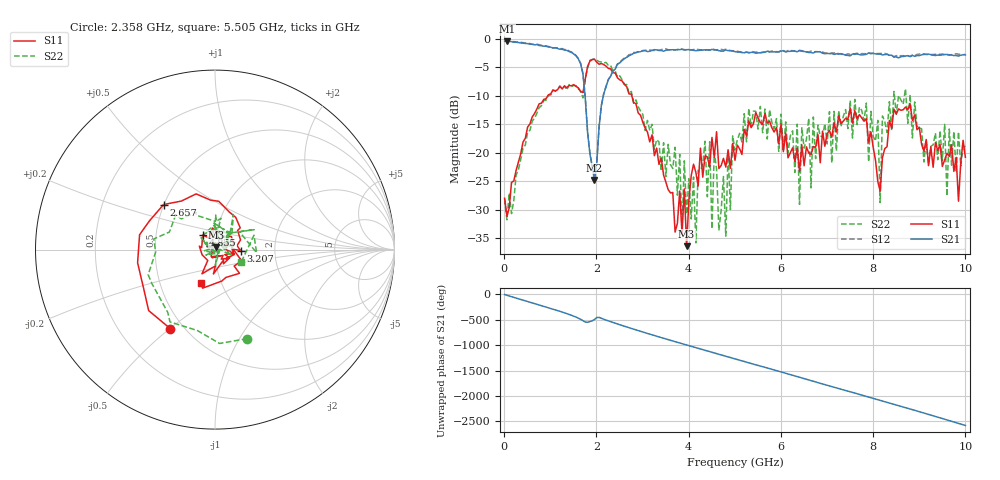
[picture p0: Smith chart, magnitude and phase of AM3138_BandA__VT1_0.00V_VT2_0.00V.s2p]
! Date/Time: Tue, Nov 13, 2018 4:41 PM
! Network Analyzer: Agilent Technologies E8364B Rev: A.07.50.67
! Sweep from 0.010 to 10.000 GHz, 201 Points, Sweep Type: LIN
! Power Supply: -0.000 V, 0.000 A
# Hz S DB R 50
!freq MagS11 AngS11 MagS21 AngS21 MagS12 AngS12 MagS22 AngS22
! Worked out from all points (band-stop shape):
!   201 points, 10 MHz to 10 GHz, reference 50 ohm
!   highest |S21| = -0.37 dB at 59.95 MHz (marker M1); lowest = -24.8 dB at 1.958 GHz (marker M2)
!   |S21| within 3 dB of the highest: start of sweep to 1.598 GHz; 2.625 GHz to end of sweep
!   lowest |S11| = -36.4 dB at 3.956 GHz (marker M3), VSWR 1.03, Z = 50.8 + j1.3 ohm
!   |S11| at or under -10 dB: start of sweep to 944.6 MHz; 2.768 GHz to end of sweep
!   |S22| runs from -35.8 to -3.5 dB; largest |S21 - S12| = 0.032
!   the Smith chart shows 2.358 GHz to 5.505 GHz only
!   S11 on the Smith chart (normalised r, x): 2.358 GHz: 0.42, -0.50; 2.657 GHz: 0.50, +0.29; 3.207 GHz: 1.34, -0.02; 4.855 GHz: 0.86, +0.14; 5.505 GHz: 0.80, -0.32
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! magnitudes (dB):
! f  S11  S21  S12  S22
! 10 MHz  -28.0  -0.4  -0.3  -28.1
! 59.95 MHz  -31.1  -0.4  -0.3  -31.8
! 1.708 GHz  -9.4  -6.1  -6.0  -10.3
! 1.958 GHz  -3.6  -24.8  -24.7  -3.5
! 2.358 GHz  -5.9  -5.6  -5.6  -5.6
! 2.657 GHz  -8.4  -3.2  -3.1  -8.0
! 3.207 GHz  -16.8  -2.0  -2.0  -15.0
! 3.357 GHz  -22.0  -2.0  -1.9  -18.1
! 3.956 GHz  -36.4  -1.9  -1.9  -30.8
! 4.456 GHz  -22.5  -2.0  -1.9  -18.1
! 4.506 GHz  -17.3  -1.8  -1.7  -33.4
! 4.805 GHz  -22.5  -1.9  -1.8  -34.6
! 4.855 GHz  -19.5  -2.0  -1.9  -19.9
! 5.005 GHz  -21.3  -2.2  -2.0  -19.5
! 5.505 GHz  -13.8  -2.4  -2.3  -15.8
! 6.354 GHz  -19.2  -2.2  -2.3  -15.0
! 6.404 GHz  -23.3  -2.0  -2.0  -29.1
! 6.703 GHz  -18.9  -2.5  -2.3  -13.7
! 7.852 GHz  -14.0  -2.7  -2.6  -11.3
! 8.152 GHz  -26.7  -2.6  -2.5  -28.8
! 8.352 GHz  -14.3  -2.8  -2.9  -11.0
! 10 GHz  -20.8  -2.8  -2.7  -19.0
